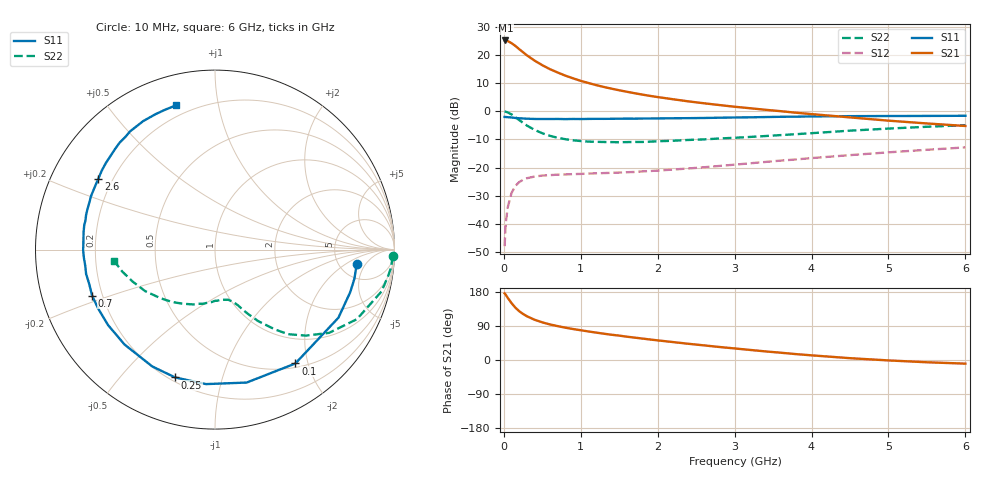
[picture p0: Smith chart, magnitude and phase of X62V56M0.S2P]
! SIEMENS Small Signal Semiconductors
! BFP193W
! Si NPN RF Bipolar Junction Transistor in SOT343
! VCE = 2.5 V  IC = 6 mA
! Common Emitter S-Parameters:  April 1994
# GHz  S  MA  R  50
!  f  S11  S21  S12  S22
! GHz  MAG  ANG  MAG  ANG  MAG  ANG  MAG  ANG
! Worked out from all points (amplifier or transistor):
!   40 points, 10 MHz to 6 GHz, reference 50 ohm
!   highest |S21| = 25.2 dB at 20 MHz (marker M1)
!   |S21| within 3 dB of that: start of sweep to 195.9 MHz
!   unconditionally stable (mu >= 1): 1.569 GHz to 4.268 GHz
!   at 200 MHz: K = 0.16, MSG = 23.6 dB, |S12| = -25.2 dB
!   at 1.5 GHz: K = 0.97, MSG = 14.6 dB, |S12| = -21.8 dB
!   at 6 GHz: K = 0.93, MSG = 3.8 dB, |S12| = -12.8 dB
!   lowest NFmin = 1.20 dB at 450 MHz
!   S11 on the Smith chart (normalised r, x): 10 MHz: 7.31, -3.18; 100 MHz: 0.56, -1.79; 250 MHz: 0.22, -0.71; 700 MHz: 0.16, -0.18; 2.6 GHz: 0.15, +0.27; 6 GHz: 0.14, +0.76
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0.01  0.7941 -5.8  18.14 175.9  0.004 88.2  0.9915 -2.1
0.02  0.7934 -11.8  18.18 173.6  0.008 84.4  0.9856 -5.9
0.03  0.7899 -17.5  18.11 170.5  0.0117 82.2  0.9761 -8.6
0.05  0.7854 -28.9  17.75 164.2  0.0195 74.9  0.9567 -14.1
0.1  0.7765 -54.8  16.28 150.1  0.0353 63.5  0.8807 -26.1
0.15  0.7615 -76.6  14.54 138.1  0.0472 53.8  0.7872 -36.1
0.2  0.751 -93.8  12.73 128.8  0.0551 46.2  0.6975 -43.4
0.25  0.7461 -107.3  11.22 121.5  0.0608 40.4  0.6235 -49.1
0.3  0.7389 -118.2  9.891 115.4  0.0646 36.4  0.5581 -53.0
0.4  0.7306 -133.6  7.96 106.2  0.0692 30.7  0.4666 -58.8
0.5  0.7292 -144.8  6.601 99.3  0.072 27.5  0.4074 -62.5
0.6  0.729 -153.0  5.609 93.8  0.0733 25.5  0.3664 -65.4
0.7  0.7312 -159.5  4.893 89.4  0.0748 24.6  0.338 -67.4
0.9  0.7308 -169.3  3.854 81.7  0.0765 23.9  0.3051 -71.5
1.1  0.732 -176.5  3.185 75.3  0.0781 24.5  0.289 -75.2
1.6  0.741 169.4  2.225 61.5  0.0826 28.7  0.2833 -85.1
2.2  0.7523 156.5  1.638 47.3  0.0921 34.8  0.2994 -98.3
2.6  0.7607 148.7  1.39 38.6  0.1011 38.1  0.3164 -107.4
3.2  0.7816 138.2  1.134 26.6  0.1189 41.4  0.3503 -120.6
4.5  0.8201 119.2  0.779 4.8  0.1663 41.1  0.4528 -149.3
5.5  0.8275 109.6  0.608 -6.0  0.2069 37.2  0.531 -166.7
6  0.8325 105.1  0.548 -9.6  0.2283 34.9  0.5657 -173.6
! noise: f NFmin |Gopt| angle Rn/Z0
0.45  1.2  0.25  114  0.13
0.9  1.25  0.37  150  0.12
1.8  2  0.55  -158  0.12
